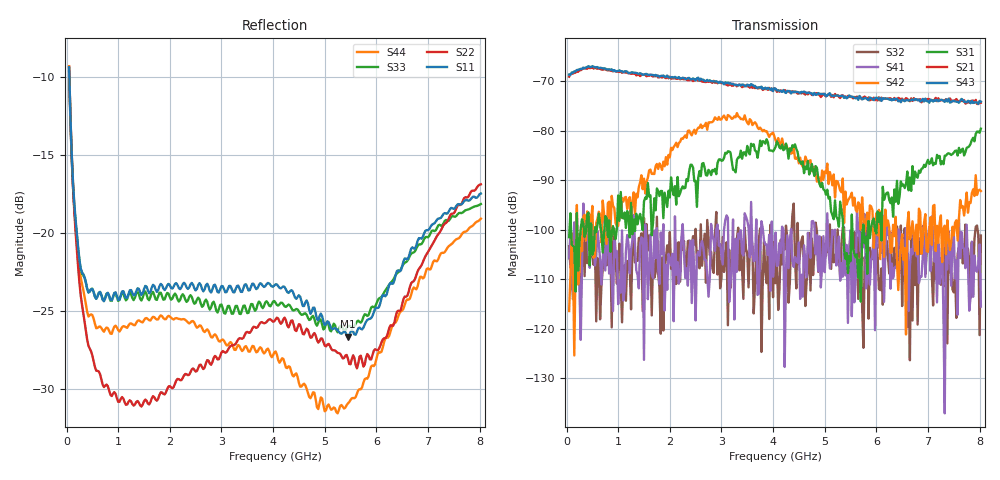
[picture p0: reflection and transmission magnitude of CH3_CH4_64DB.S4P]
!Agilent Technologies,E5071C,MY46316741,A.11.02
!Date: Thu May 28 15:01:08 2026
!Data & Calibration Information:
!1:CH3 INPUT 2:CH3 OUTPUT 3:CH4 INPUT 4:CH4 OUTPUT
!Freq	S11:SOLT4(ON)	S12:SOLT4(ON)	S13:SOLT4(ON)	S14:SOLT4(ON)
!	S21:SOLT4(ON)	S22:SOLT4(ON)	S23:SOLT4(ON)	S24:SOLT4(ON)
!	S31:SOLT4(ON)	S32:SOLT4(ON)	S33:SOLT4(ON)	S34:SOLT4(ON)
!	S41:SOLT4(ON)	S42:SOLT4(ON)	S43:SOLT4(ON)	S44:SOLT4(ON)
!PortZ  Port1:50+j0  Port2:50+j0  Port3:50+j0  Port4:50+j0
!Above PortZ is port z conversion or system Z0 setting when saving the data.
!When reading, reference impedance value at option line is always used.
# Hz S dB R 50
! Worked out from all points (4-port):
!   320 points, 50 MHz to 8.025 GHz, reference 50 ohm
!   strongest paths, dB at 50 MHz, 2.05 GHz, 4.05 GHz, 6.05 GHz, 8.025 GHz:
!     S43: -68.7, -69.2, -71.5, -73.7, -74.1
!     S21: -69.1, -69.4, -71.6, -73.3, -74.3
!     S31: -101.5, -91.9, -83.2, -98.5, -79.6
!     S42: -116.4, -83.9, -82.0, -96.0, -92.2
!     S41: -105.8, -104.8, -100.6, -103.6, -115.5
!     S32: -103.3, -106.3, -110.8, -111.9, -101.2
!   lowest |S11| = -26.7 dB at 5.45 GHz (marker M1), VSWR 1.10, Z = 48 - j4.11 ohm
!   |S11| at or under -10 dB: 55.14 MHz to end of sweep
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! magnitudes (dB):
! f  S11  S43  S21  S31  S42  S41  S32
! 50 MHz  -9.3  -68.7  -69.1  -101.5  -116.4  -105.8  -103.3
! 125 MHz  -16.7  -68.3  -68.5  -103.3  -105.5  -112.5  -114.0
! 275 MHz  -22.3  -67.5  -67.8  -99.7  -101.4  -122.2  -113.7
! 850 MHz  -24.3  -67.7  -67.9  -104.4  -100.6  -102.6  -102.2
! 3.3 GHz  -23.4  -70.8  -71.0  -85.9  -76.4  -108.5  -101.7
! 5.45 GHz  -26.7  -73.3  -73.0  -108.7  -94.1  -118.8  -105.3
! 8.025 GHz  -17.5  -74.1  -74.3  -79.6  -92.2  -115.5  -101.2
